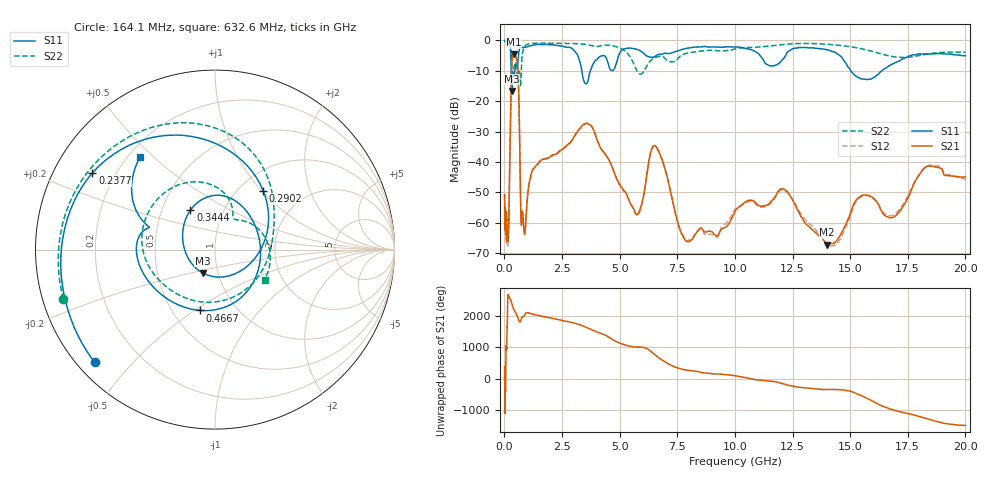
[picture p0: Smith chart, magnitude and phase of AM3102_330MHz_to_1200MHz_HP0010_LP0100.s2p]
! Date/Time: Tue, Sep 11, 2018 5:10 PM
! Network Analyzer: Agilent Technologies E8362B Rev: A.07.50.63
! Sweep from 0.010 to 20.000 GHz, 1601 Points, Sweep Type: LOG
! Power Supply: 4.949 V, 0.001 A
# Hz S DB R 50
!freq MagS11 AngS11 MagS21 AngS21 MagS12 AngS12 MagS22 AngS22
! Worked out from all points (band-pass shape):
!   1601 points, 10 MHz to 20 GHz, reference 50 ohm
!   highest |S21| = -4.54 dB at 412.5 MHz (marker M1); lowest = -67.2 dB at 14.01 GHz (marker M2)
!   |S21| within 3 dB of the highest: 324 MHz to 570.1 MHz (246.1 MHz wide, 55 % of centre)
!   lowest |S11| = -16.7 dB at 319.2 MHz (marker M3), VSWR 1.34, Z = 42.2 - j11.2 ohm
!   |S11| at or under -10 dB: 297.7 MHz to 447.9 MHz (150.3 MHz wide, 40.3 % of centre); 3.36 GHz to 3.733 GHz (373.3 MHz wide, 10.5 % of centre); 15.03 GHz to 16.37 GHz (1.346 GHz wide, 8.58 % of centre)
!   |S22| runs from -15.2 to -0.2 dB; largest |S21 - S12| = 0.011
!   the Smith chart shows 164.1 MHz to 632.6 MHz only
!   S11 on the Smith chart (normalised r, x): 164.1 MHz: 0.05, -0.39; 237.7 MHz: 0.12, +0.28; 290.2 MHz: 1.28, +1.02; 344.4 MHz: 0.70, +0.33; 466.7 MHz: 0.68, -0.53; 632.6 MHz: 0.25, +0.45
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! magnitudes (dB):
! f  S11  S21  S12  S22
! 10 MHz  0.0  -50.9  -50.5  -0.2
! 35.55 MHz  0.0  -60.9  -61.3  -0.4
! 126.4 MHz  -0.4  -65.6  -63.9  -0.8
! 164.1 MHz  -0.7  -64.4  -65.5  -1.0
! 237.7 MHz  -1.9  -39.0  -39.1  -1.8
! 290.2 MHz  -7.5  -15.9  -15.9  -4.0
! 319.2 MHz  -16.7  -8.2  -8.2  -7.8
! 344.4 MHz  -11.7  -5.9  -6.0  -10.5
! 412.5 MHz  -11.9  -4.5  -4.6  -9.3
! 447.2 MHz  -10.0  -4.8  -4.8  -7.9
! 466.7 MHz  -9.1  -5.0  -5.0  -7.5
! 632.6 MHz  -3.6  -20.6  -20.7  -9.8
! 726 MHz  -2.2  -59.6  -60.1  -11.7
! 869.7 MHz  -2.2  -63.5  -63.8  -2.0
! 1.59 GHz  -1.4  -39.4  -39.5  -0.9
! 3.651 GHz  -12.4  -27.6  -27.3  -1.5
! 5.652 GHz  -2.7  -56.2  -56.4  -8.4
! 6.549 GHz  -5.2  -34.7  -34.9  -5.6
! 7.882 GHz  -2.6  -66.1  -65.8  -4.3
! 12.03 GHz  -6.6  -48.8  -49.3  -1.4
! 14.01 GHz  -3.1  -67.2  -67.2  -1.3
! 20 GHz  -5.0  -45.0  -45.7  -3.8
